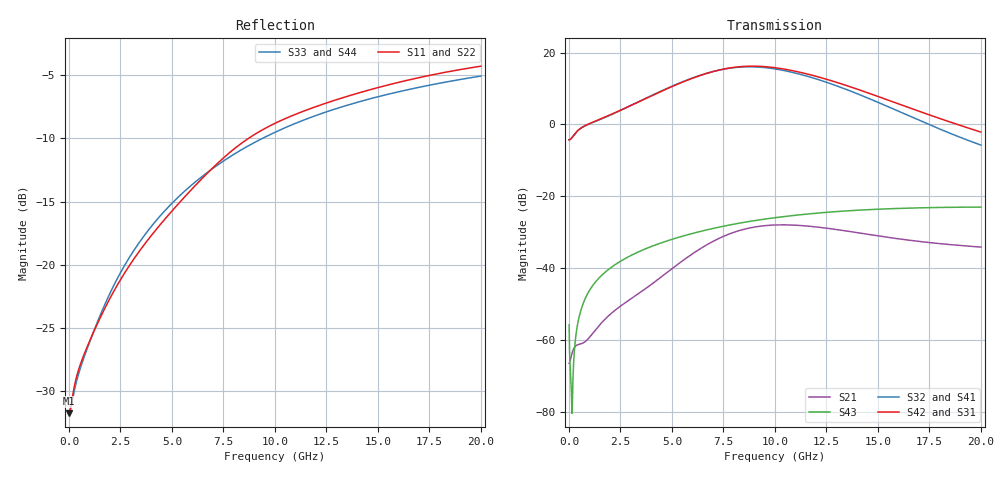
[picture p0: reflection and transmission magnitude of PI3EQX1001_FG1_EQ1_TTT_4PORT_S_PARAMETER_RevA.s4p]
! NPort=4 DATA=2000 NOISE=0 GROUPDELAY=0 COMPLEX_DATAFORMAT=POLAR
! NumOfBlock=1 NumOfParam=0
! .MODEL Smodel S TSTONEFILE=PI3EQX1001_FG1_EQ1_TTT_4PORT_S_PARAMETER_RevA.s4p TYPE=S
!  -- The above .MODEL line can be used for the S element in the netlist.
! The s parameter is extracted from the linear redriver, it is not bi-directional; only s(4,1)s(4,2) and s(3,1)s(3,2)
! should be the insertion loss
!Port definition:
!Port1 = input+
!Port2 = input¨C
!Port3 = output+
!Port4 = output-
# Hz S MA R  50
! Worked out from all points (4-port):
!   2000 points, 10 MHz to 20 GHz, reference 50 ohm
!   strongest paths, dB at 10 MHz, 5.01 GHz, 10.01 GHz, 15.01 GHz, 20 GHz:
!     S42: -4.3, 10.6, 15.8, 7.8, -2.1
!     S31: -4.3, 10.6, 15.8, 7.8, -2.1
!     S32: -4.3, 10.7, 15.5, 6.1, -5.7
!     S41: -4.3, 10.6, 15.4, 6.1, -5.8
!     S43: -55.8, -32.0, -26.0, -23.6, -23.0
!     S21: -66.5, -40.1, -28.0, -31.0, -34.1
!   lowest |S11| = -31.7 dB at 10 MHz (marker M1), VSWR 1.05, Z = 47.5 - j0.063 ohm
!   |S11| at or under -10 dB: start of sweep to 8.712 GHz
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1e7  0.02591 -178.5  0.0004939 2.7  3.669e-05 -0.2  4.787e-05 -0.1
     0.0004742 2.9  0.02597 -178.7  4.577e-05 -0.2  5.994e-05 -0.1
     0.6121 0.3  0.6121 -179.7  0.02616 178.4  0.001614 -59.2
     0.6118 -179.7  0.6118 0.3  0.001627 -58.9  0.02612 178.4
5.94e9  0.1982 -104.7  0.01475 102.6  2.35e-05 -30.6  3.338e-05 -28.9
        0.01543 101.1  0.1967 -104.6  3.063e-05 -26.5  4.236e-05 -24.3
        4.333 -47.6  4.371 135.1  0.2064 -111.1  0.03013 61.9
        4.358 135.1  4.332 -47.5  0.03011 61.8  0.2062 -111.0
8.01e9  0.287 -106.5  0.03041 70.4  2.062e-05 -28.7  3.15e-05 -30.9
        0.03157 69.1  0.2854 -106.5  2.928e-05 -26.0  3.948e-05 -24.5
        6.223 -108.2  6.171 74.6  0.2738 -113.2  0.04107 49.6
        6.145 74.6  6.228 -108.0  0.04096 49.5  0.2736 -113.1
9.98e9  0.3621 -112.1  0.03855 33.1  2.163e-05 -23.9  3.221e-05 -37.0
        0.03987 31.8  0.3596 -112.2  3.05e-05 -31.0  4.011e-05 -24.3
        6.167 -171.4  5.943 11.6  0.3337 -116.1  0.0505 36.9
        5.914 11.7  6.173 -171.3  0.05028 36.9  0.3337 -116.1
1.256e10  0.4382 -118.0  0.03474 -3.5  2.726e-05 -35.6  3.085e-05 -55.0
          0.03585 -4.7  0.4346 -118.1  2.927e-05 -47.3  4.462e-05 -33.5
          4.204 115.8  3.815 -60.5  0.4043 -120.4  0.06013 20.4
          3.794 -60.3  4.208 115.8  0.05999 20.5  0.4042 -120.4
1.523e10  0.5081 -122.9  0.02666 -24.0  2.721e-05 -66.0  2.385e-05 -81.9
          0.02755 -25.1  0.5038 -123.0  2.211e-05 -71.0  4.209e-05 -54.4
          2.323 55.9  1.905 -118.1  0.4672 -124.6  0.06655 4.0
          1.893 -117.7  2.325 56.0  0.06653 4.1  0.4667 -124.5
2e10  0.6105 -131.1  0.019 -36.8  1.242e-05 -153.9  9.995e-06 152.5
      0.01964 -38.4  0.6051 -131.2  6.059e-06 134.1  1.521e-05 -92.6
      0.7833 -19.6  0.5162 -177.7  0.5579 -131.2  0.07071 -23.1
      0.5136 -176.9  0.7828 -19.4  0.0707 -23.2  0.5578 -131.1
